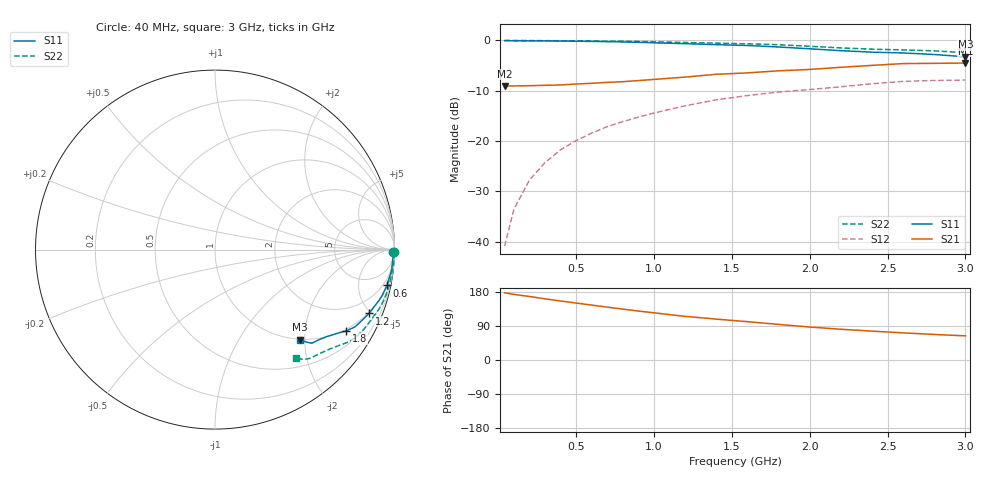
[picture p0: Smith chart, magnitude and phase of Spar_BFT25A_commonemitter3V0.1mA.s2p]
! Filename:  BFT25AF.S2P  Version:  2.0
! NXP part #: BFT25A  Date: Aug 1990
! Bias condition: Vce=3V, Ic=0.1mA
#  MHz  S  MA  R  50
! Freq  S11  S21  S12  S22  !GUM [dB]
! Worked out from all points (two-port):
!   21 points, 40 MHz to 3 GHz, reference 50 ohm
!   highest |S21| = -4.50 dB at 3 GHz (marker M1); lowest = -9.1 dB at 40 MHz (marker M2)
!   |S21| within 3 dB of the highest: 1.11 GHz to end of sweep
!   lowest |S11| = -3.2 dB at 3 GHz (marker M3), VSWR 5.41, Z = 49.6 - j94.4 ohm
!   |S11| at or under -10 dB: nowhere
!   |S22| runs from -2.4 to 0.0 dB; largest |S21 - S12| = 0.35
!   S11 on the Smith chart (normalised r, x): 40 MHz: open; 600 MHz: 1.04, -9.56; 1.2 GHz: 0.94, -4.85; 1.8 GHz: 0.94, -3.28; 3 GHz: 0.99, -1.89
40  0.994 -0.9  0.352 177.4  0.009 88.7  1 -0.9
100  0.993 -2.0  0.353 173.1  0.021 87.2  0.999 -2.2
200  0.991 -4.0  0.355 167.6  0.041 85.9  0.997 -4.3
300  0.991 -6.0  0.358 161.4  0.061 84.5  0.995 -6.4
400  0.987 -7.9  0.361 155.7  0.082 82.6  0.993 -8.6
500  0.982 -9.7  0.369 150.3  0.101 81.1  0.992 -10.7
600  0.978 -11.8  0.375 144.8  0.12 79.6  0.989 -12.7
700  0.972 -13.5  0.383 139.5  0.139 77.9  0.986 -14.7
800  0.967 -15.2  0.389 134.3  0.156 76.1  0.982 -16.6
900  0.958 -17.0  0.399 129.1  0.173 74.3  0.977 -18.5
1000  0.948 -18.7  0.41 124.5  0.19 72.5  0.97 -20.4
1200  0.929 -22.5  0.432 115.1  0.224 68.6  0.954 -24.2
1400  0.908 -25.9  0.461 107.9  0.257 65.5  0.941 -28.0
1600  0.891 -28.9  0.476 101.1  0.283 62.4  0.926 -31.3
1800  0.861 -31.7  0.499 93.9  0.307 59.4  0.907 -34.5
2000  0.826 -34.4  0.515 87.0  0.325 55.3  0.875 -37.5
2200  0.791 -37.7  0.541 81.1  0.346 51.5  0.843 -41.3
2400  0.765 -41.2  0.565 76.2  0.371 48.5  0.819 -45.4
2600  0.751 -44.0  0.589 71.6  0.392 45.8  0.805 -48.8
2800  0.725 -45.3  0.592 67.4  0.4 43.9  0.788 -51.0
3000  0.688 -46.8  0.596 63.7  0.404 41.5  0.756 -53.2
